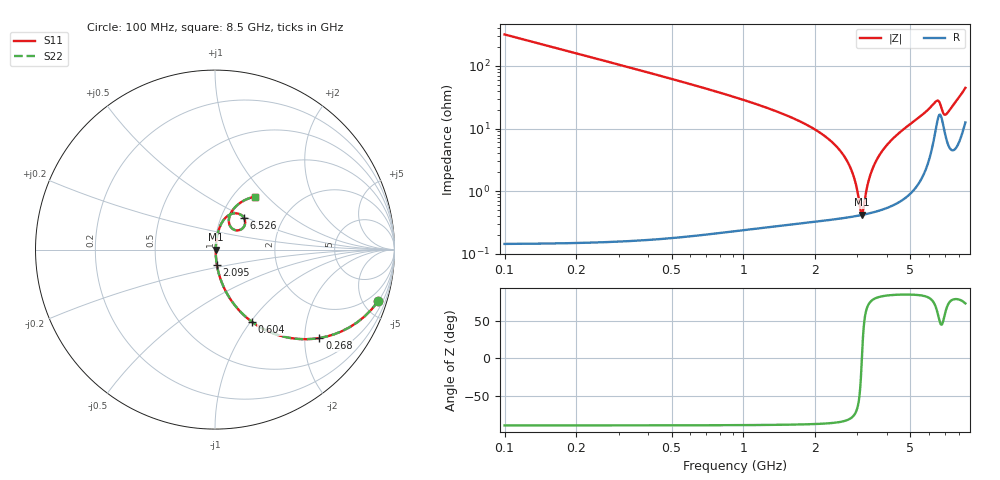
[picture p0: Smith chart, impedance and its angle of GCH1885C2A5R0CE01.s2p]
!Murata Part Number: GCH1885C2A5R0CE01
!These Parameters are Measured in Series Mode Connection
!Data Generated on Mar 13, 2026
!  o--ll--o
!Port1  Port2
!  o------o
!Operation Temp=25[degC], DC Bias Voltage=0[V]
!Freq. Start=100[MHz] Stop=9[GHz] 401[Steps]
# Hz S RI R 50
!Freq.(Hz) S11(Real) S11(Imag) S21(Real) S21(Imag) S12(Real) S12(Imag) S22(Real) S22(Imag)
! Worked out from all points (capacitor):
!   401 points, 100 MHz to 8.5 GHz, reference 50 ohm
!   read as one part in series: C = 5 pF near 142 MHz
!   lowest |Z| = 420 mohm at 3.124 GHz (marker M1)
!   series resonance near 3.133 GHz, so ESL is about 520 pH
!   S11 on the Smith chart (normalised r, x): 100 MHz: 1.00, -6.36; 268 MHz: 1.00, -2.36; 604 MHz: 1.00, -1.02; 2.095 GHz: 1.01, -0.17; 6.526 GHz: 1.29, +0.48; 8.5 GHz: 1.25, +0.86
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1e8  0.9099 -0.2861  0.0901 0.2861  0.0901 0.2861  0.9099 -0.2861
2.68e8  0.5815 -0.4927  0.4185 0.4927  0.4185 0.4927  0.5815 -0.4927
4.15e8  0.3625 -0.4796  0.6375 0.4796  0.6375 0.4796  0.3625 -0.4796
6.04e8  0.2058 -0.4024  0.7942 0.4024  0.7942 0.4024  0.2058 -0.4024
9.4e8  0.0887 -0.2806  0.9113 0.2806  0.9113 0.2806  0.0887 -0.2806
1.507e9  0.0287 -0.1584  0.9713 0.1584  0.9713 0.1584  0.0287 -0.1584
2.095e9  0.0105 -0.0843  0.9895 0.0843  0.9895 0.0843  0.0105 -0.0843
2.599e9  0.0052 -0.039  0.9948 0.039  0.9948 0.039  0.0052 -0.039
2.788e9  0.00442 -0.0244  0.9956 0.0244  0.9956 0.0244  0.00442 -0.0244
2.914e9  0.00417 -0.0152  0.9958 0.0152  0.9958 0.0152  0.00417 -0.0152
3.124e9  0.00413 -0.000607  0.9959 0.000607  0.9959 0.000607  0.00413 -0.000607
3.166e9  0.00418 0.00222  0.9958 -0.00222  0.9958 -0.00222  0.00418 0.00222
3.355e9  0.0046 0.0146  0.9954 -0.0146  0.9954 -0.0146  0.0046 0.0146
3.544e9  0.00533 0.0266  0.9947 -0.0266  0.9947 -0.0266  0.00533 0.0266
3.859e9  0.00722 0.0458  0.9928 -0.0458  0.9928 -0.0458  0.00722 0.0458
4.3e9  0.0113 0.072  0.9887 -0.072  0.9887 -0.072  0.0113 0.072
5.707e9  0.0466 0.163  0.9534 -0.163  0.9534 -0.163  0.0466 0.163
6.526e9  0.1626 0.1741  0.8374 -0.1741  0.8374 -0.1741  0.1626 0.1741
6.883e9  0.1104 0.1091  0.8896 -0.1091  0.8896 -0.1091  0.1104 0.1091
7.114e9  0.0803 0.1401  0.9197 -0.1401  0.9197 -0.1401  0.0803 0.1401
7.807e9  0.1088 0.2326  0.8912 -0.2326  0.8912 -0.2326  0.1088 0.2326
8.5e9  0.2239 0.2958  0.7761 -0.2958  0.7761 -0.2958  0.2239 0.2958
